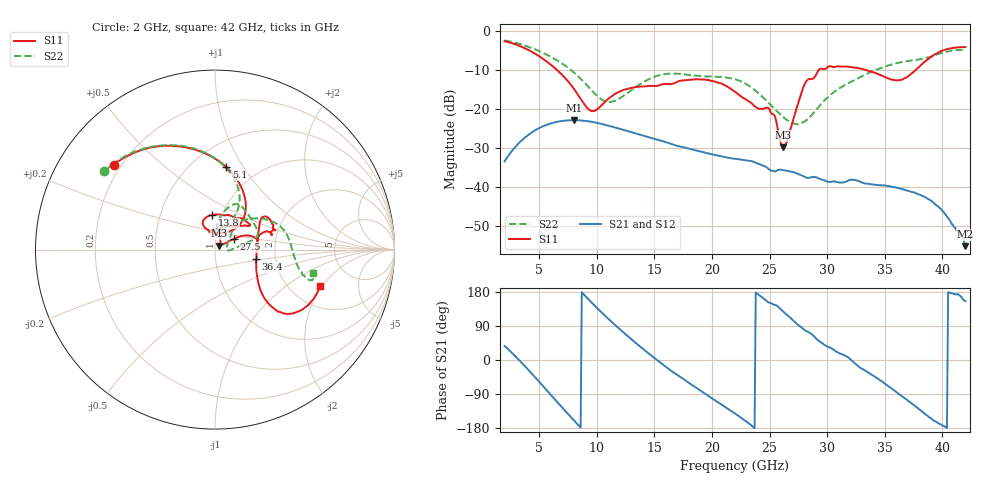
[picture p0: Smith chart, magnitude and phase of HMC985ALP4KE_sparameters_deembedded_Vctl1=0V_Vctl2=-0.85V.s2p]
!s2p File: Measurements: S11, S21, S12, S22
# GHz S dB R 50.0
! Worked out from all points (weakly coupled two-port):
!   401 points, 2 GHz to 42 GHz, reference 50 ohm
!   highest |S21| = -22.89 dB at 8 GHz (marker M1); lowest = -55.2 dB at 42 GHz (marker M2)
!   lowest |S11| = -29.8 dB at 26.2 GHz (marker M3), VSWR 1.07, Z = 52.4 + j2.25 ohm
!   |S11| at or under -10 dB: 6.544 GHz to 29.27 GHz (22.73 GHz wide, 127 % of centre); 33.35 GHz to 37.69 GHz (4.344 GHz wide, 12.2 % of centre)
!   |S22| runs from -23.9 to -2.4 dB; largest |S21 - S12| = 0.00017
!   S11 on the Smith chart (normalised r, x): 2 GHz: 0.17, +0.35; 5.1 GHz: 0.72, +0.84; 13.8 GHz: 0.90, +0.36; 27.5 GHz: 1.22, +0.15; 36.4 GHz: 1.58, -0.17; 42 GHz: 2.91, -1.91
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2  -2.65 140.0  -33.45 37.0  -33.45 37.0  -2.45 144.7
3.5  -4.10 112.2  -28.03 -7.8  -28.04 -7.8  -3.51 120.5
5.1  -6.69 82.1  -24.76 -60.9  -24.77 -60.9  -5.31 96.0
8  -14.78 45.5  -22.89 -158.8  -22.89 -158.8  -10.61 62.5
8.7  -17.87 51.7  -22.98 178.6  -22.98 178.6  -12.56 59.7
9.7  -20.57 86.0  -23.38 147.2  -23.38 147.2  -15.69 62.3
11  -17.40 114.6  -24.28 108.7  -24.28 108.7  -18.20 77.1
13.8  -14.27 95.3  -26.64 34.6  -26.64 34.6  -13.58 77.5
15.4  -13.94 73.0  -28.01 -3.8  -28.01 -3.8  -11.38 68.3
19.4  -12.52 34.6  -31.21 -88.9  -31.22 -89.0  -11.65 35.7
22  -15.60 52.2  -32.78 -141.1  -32.79 -141.2  -12.39 16.5
25  -20.20 97.8  -35.61 150.9  -35.62 150.8  -18.74 5.0
26.2  -29.82 41.6  -35.70 127.4  -35.72 127.3  -22.12 -3.2
27.5  -18.40 29.7  -36.72 92.1  -36.68 92.0  -23.82 4.3
28.1  -13.36 20.7  -37.48 77.9  -37.48 77.8  -23.13 17.2
28.7  -12.31 12.8  -37.45 66.8  -37.45 67.1  -21.44 29.4
31  -9.09 23.3  -38.83 19.0  -38.86 19.1  -14.80 49.8
33.3  -9.96 34.4  -39.11 -28.2  -39.11 -28.2  -11.26 39.2
35.4  -12.27 12.4  -39.81 -71.2  -39.84 -71.3  -8.79 24.4
36.4  -12.57 -12.8  -40.48 -93.6  -40.48 -93.6  -8.01 16.3
39.5  -5.80 -43.3  -44.73 -163.6  -44.69 -164.0  -6.05 -14.7
42  -4.14 -19.0  -55.19 155.1  -55.27 152.7  -4.98 -13.6
